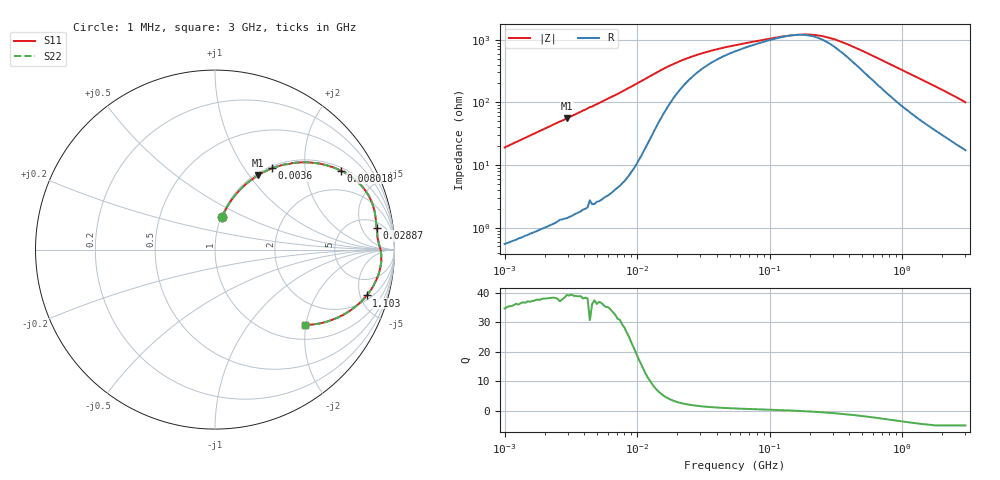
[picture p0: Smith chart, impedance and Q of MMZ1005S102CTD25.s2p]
! S-Parameter Data Generated by TDK Corporation
! Copyright(C) 2025 TDK Corporation.
! All Rights Reserved.
! TDK P/N: MMZ1005S102CTD25 (Chip Bead)
! Property: |Z|=1000ohm at 100MHz
! Size(LxWxT): 1x0.5x0.5mm
! Model Type: s2p (Touchstone File Format Version 1.0)
! Frequency: DC=Yes Start=1MHz Stop=3000MHz 202points Log-sweep
! Model Generated on Feb. 6, 2025
! Terms and conditions regarding TDK Simulation Models:
! 1)This simulation model is being provided solely for informational
!  purposes. Please refer to the specifications of the products in
!  terms of detailed characteristics of such products.
! 2)In no event shall TDK Corporation of any of its subsidiaries be
!  liable for any loss or damage arising, directly or indirectly,
!  from any information contained in this simulation model, including,
!  but not limited to loss or damages arising from any inaccuracies,
!  omissions or errors in connection with such information.
! 3)Any and all copyrights on this simulation model are owned by
!  TDK Corporation.  Duplication or redistribution of this simulation
!  model without prior written permission from TDK Corporation
!  is prohibited.
! 4)This simulation model is subject to any modification or change
!  without any prior notice.
! 5)Neither TDK Corporation nor any of its subsidiaries shall make any
!  warranty, express or implied, including but not limited to the
!  correctness, implied warranties of merchantability and fitness for
!  a particular purpose with respect to this simulation models.
! 6)The use of this simulation model shall be deemed to have consented
!  to the terms and conditions hereof.
! Port Assignments:
!  1 ---@@@--- 2
! Applicable Conditions:
!  Temperature = 25 degC
!  DC Bias Current = 0 A
!  Small Signal Operation
# Hz S MA R 50
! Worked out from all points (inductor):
!   201 points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, 1 MHz to 3 GHz, reference 50 ohm
!   read as one part in series: L = 3.02 uH near 1.041 MHz
!   highest Q = 39 at 2.947 MHz (marker M1), where L = 2.99 uH
!   self-resonance near 153.8 MHz
!   S11 on the Smith chart (normalised r, x): 1 MHz: 1.01, +0.38; 3.6 MHz: 1.03, +1.35; 8.018 MHz: 1.11, +3.11; 28.87 MHz: 7, +10; 1.103 GHz: 2.47, -5.73; 3 GHz: 1.34, -1.98
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1000000  0.1861 77.6  0.9772 -10.7  0.9772 -10.7  0.1861 77.6
1822989  0.3234 69.6  0.9377 -18.9  0.9377 -18.9  0.3234 69.6
2947212  0.4797 59.9  0.8653 -28.7  0.8653 -28.7  0.4797 59.9
3600306  0.5544 54.9  0.8181 -33.7  0.8181 -33.7  0.5544 54.9
3900413  0.5856 52.7  0.7953 -35.8  0.7953 -35.8  0.5856 52.7
5592179  0.7175 42.6  0.6768 -45.8  0.6768 -45.8  0.7175 42.6
8017732  0.8281 32.1  0.532 -55.9  0.532 -55.9  0.8281 32.1
1.104425e7  0.8918 23.2  0.395 -62.8  0.395 -62.8  0.8918 23.2
1.461624e7  0.9127 16.7  0.2905 -64.4  0.2905 -64.4  0.9127 16.7
2.013356e7  0.9124 11.4  0.2091 -59.7  0.2091 -59.7  0.9124 11.4
2.886629e7  0.9083 7.6  0.1566 -50.4  0.1566 -50.4  0.9083 7.6
5.477226e7  0.9088 3.9  0.1115 -33.2  0.1115 -33.2  0.9088 3.9
1.375402e8  0.9208 0.4  0.0796 -5.2  0.0796 -5.2  0.9208 0.4
1.820241e8  0.9245 -0.7  0.07639 8.5  0.07639 8.5  0.9245 -0.7
2.136344e8  0.9262 -1.4  0.07759 17.3  0.07759 17.3  0.9262 -1.4
2.716345e8  0.928 -2.7  0.08486 30.7  0.08486 30.7  0.928 -2.7
3.453811e8  0.9286 -4.1  0.09983 42.3  0.09983 42.3  0.9286 -4.1
8.005644e8  0.9088 -12.1  0.2204 59.7  0.2204 59.7  0.9088 -12.1
1.10276e9  0.8832 -16.8  0.2985 58.8  0.2985 58.8  0.8832 -16.8
1.782824e9  0.8088 -26.2  0.45 52.5  0.45 52.5  0.8088 -26.2
2.266846e9  0.7491 -32.1  0.5398 47.4  0.5398 47.4  0.7491 -32.1
3e9  0.654 -40.0  0.6524 40.1  0.6524 40.1  0.654 -40.0
